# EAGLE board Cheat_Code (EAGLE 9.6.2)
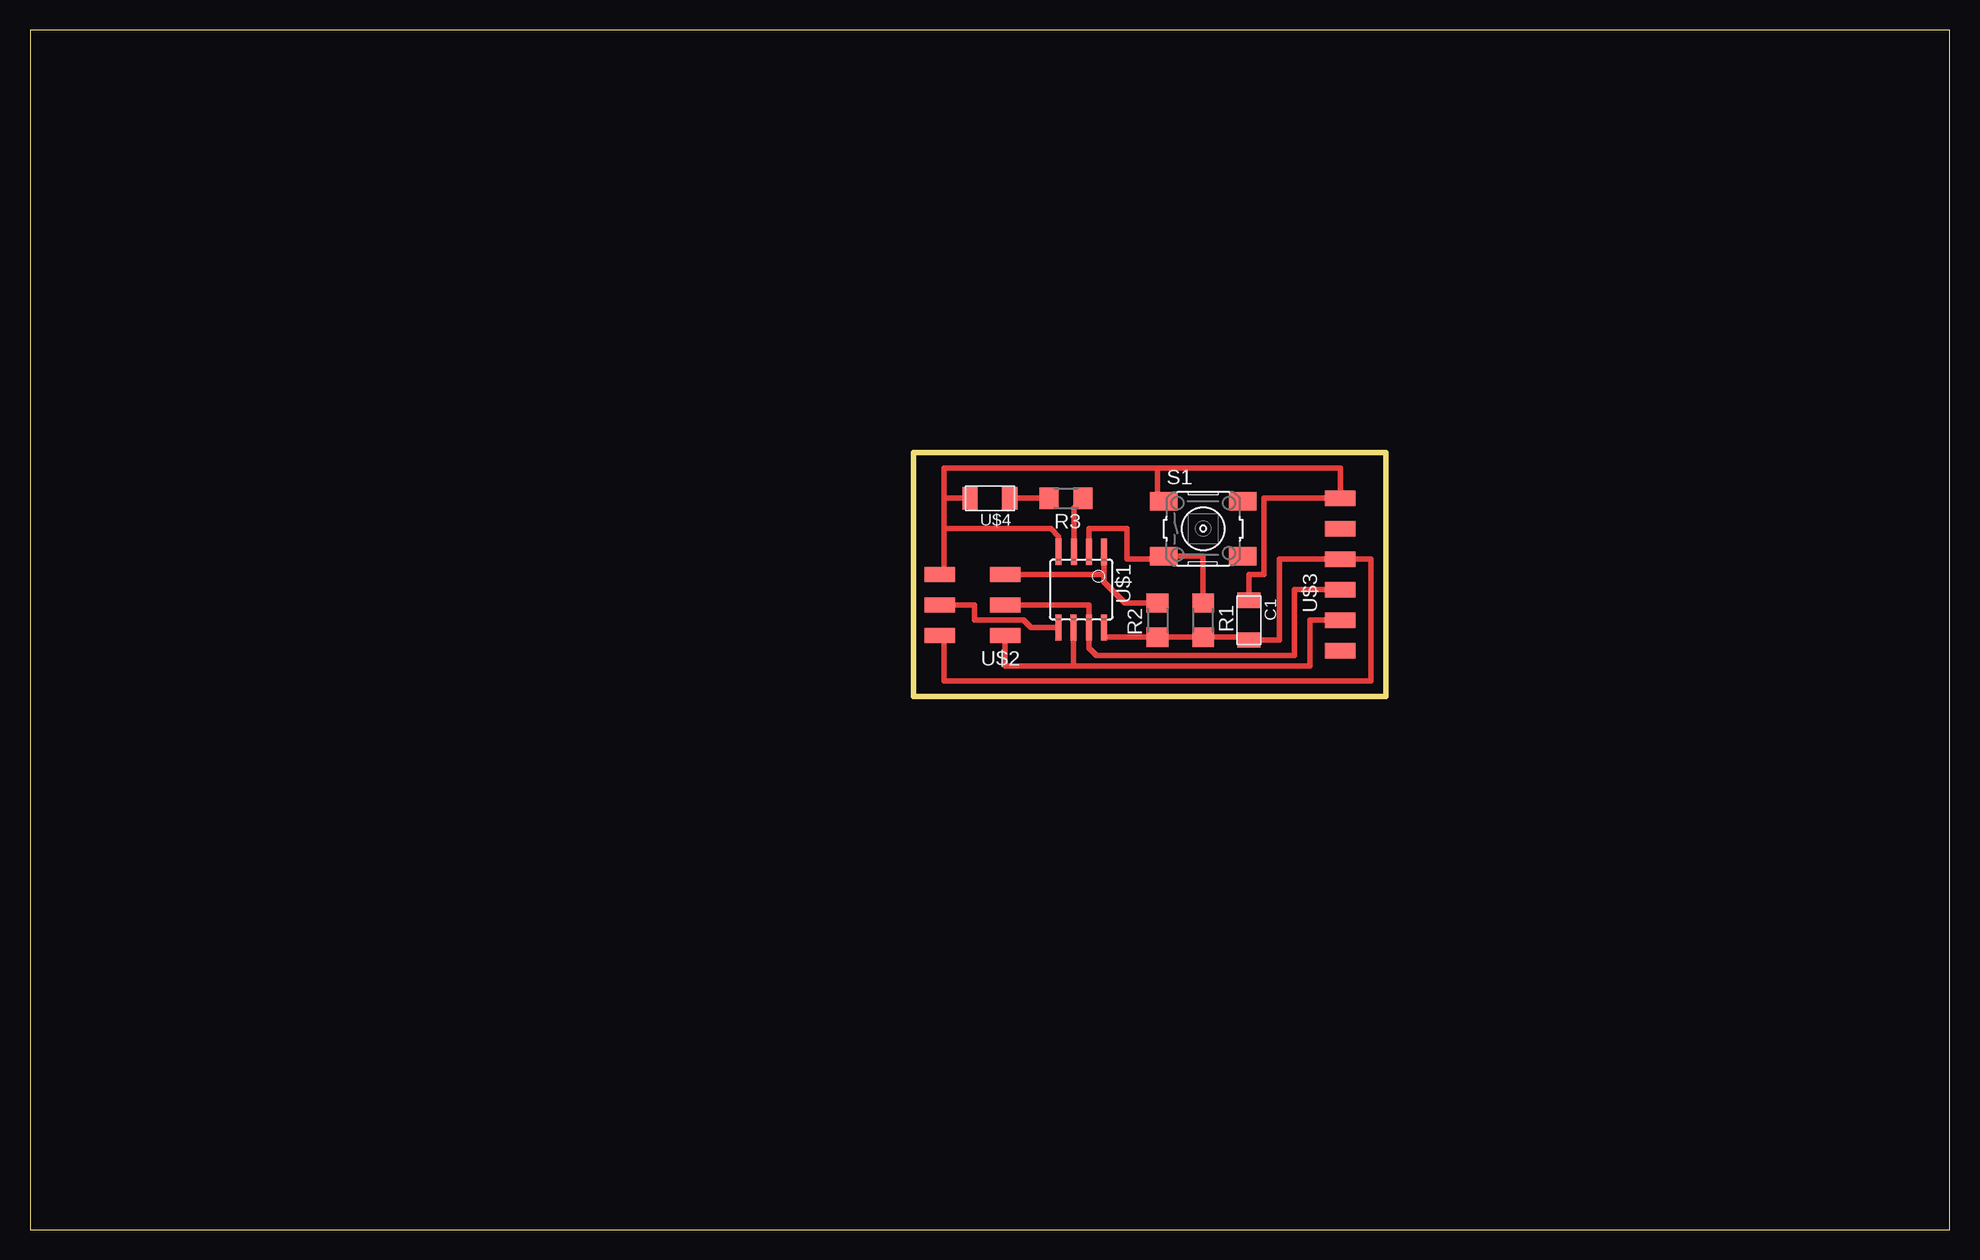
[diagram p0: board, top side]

Size 160 x 100 mm. Coordinates in mm from the lower left corner, seen from the top.
Outline: 0,0 160,0 160,100 0,100 0,0
Copper layers (1*16): Top 0.035mm / dielectric 1.5mm / Bottom 0.035mm
Design rules "default *": minimum track width 18mil, minimum drill 0.35mm, track to track 16mil, track to pad 16mil, pad to pad 16mil, via to via 12mil, smd to smd 10mil, copper to edge 40mil, drill to drill 6mil, minimum pad ring 10mil, minimum via ring 8mil, stop-mask expansion 4mil, vias tented up to drill 0mil, thermal gap 10mil
Milling: 6 lines

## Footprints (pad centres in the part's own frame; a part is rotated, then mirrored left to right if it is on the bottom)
C1206FAB = smd 1.27 x 1.905: 1 -1.651,0; 2 1.651,0
R1206 = smd 1.6 x 1.803: 1 -1.422,0; 2 1.422,0
6MM_SWITCH = smd 2.286 x 1.524: 1 -3.302,2.286; 2 3.302,2.286; 3 -3.302,-2.286; 4 3.302,-2.286
SOIC8 = smd 0.5 x 2.2: 1 -1.905,-3.154; 2 -0.645,-3.154; 3 0.625,-3.154; 4 1.895,-3.154; 5 1.905,3.154; 6 0.635,3.154; 7 -0.635,3.154; 8 -1.905,3.154
2X03SMD = smd 2.54 x 1.27: 1 -2.54,2.54; 2 2.92,2.54; 3 -2.54,0; 4 2.92,0; 5 -2.54,-2.54; 6 2.92,-2.54
1X06SMD = smd 2.54 x 1.27: 1 0,6.35; 2 0,3.81; 3 0,1.27; 4 0,-1.27; 5 0,-3.81; 6 0,-6.35
LED1206FAB = smd 1.27 x 1.905: 1 -1.651,0; 2 1.651,0

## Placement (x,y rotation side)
C1  1u  [C1206FAB]  101.6,50.8 270 top
R1  10k  [R1206]  97.79,50.8 270 top
R2  10k  [R1206]  93.98,50.8 90 top
R3  10k  [R1206]  86.36,60.96 180 top
S1  [6MM_SWITCH]  97.79,58.42 0 top
U$1  UC_ATTINY45SI  [SOIC8]  87.63,53.34 180 top
U$2  CONN_03X2_AVRISPSMD  [2X03SMD]  78.74,52.07 180 top
U$3  CONN_06_FTDI-SMD-HEADER  [1X06SMD]  109.22,54.61 0 top
U$4  LEDFAB1206  [LED1206FAB]  80.01,60.96 180 top

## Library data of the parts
C1 R1-R3 S1 U$1-U$4 = fab

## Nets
GND: C1.1 S1.1 U$1.4 U$2.6 U$3.1 U$4.2
LED: R3.1 U$1.3
N$1: U$1.6 U$2.1 U$3.5
N$2: U$1.7 U$2.3 U$3.4
N$3: R2.2 U$1.1 U$2.5
N$4: U$1.5 U$2.4
N$5: R3.2 U$4.1
PB: R1.1 S1.3 U$1.2
VCC: C1.2 R1.2 R2.1 U$1.8 U$2.2 U$3.3

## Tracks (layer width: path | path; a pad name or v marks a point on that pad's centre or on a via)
GND
  Top 0.457: 93.98,63.5 76.2,63.5 76.2,60.96 | 93.98,63.5 109.22,63.5 U$3.1 102.87,60.96 102.87,54.61 101.6,54.61 C1.1 | U$4.2 76.2,60.96 | S1.1 93.98,61.21 93.98,63.5 | U$1.4 85.73,57.77 85.09,58.42 76.2,58.42 | U$2.6 76.2,54.99 76.2,58.42 | 76.2,58.42 76.2,60.96
LED
  Top 0.457: R3.1 87,60.18 U$1.3
N$1
  Top 0.457: U$3.5 106.68,50.8 106.68,46.99 87,46.99 | 87,46.99 81.28,46.99 U$2.1 | U$1.6 87,46.99
N$2
  Top 0.457: U$3.4 105.41,53.34 105.41,47.85 88.9,47.85 88.27,48.49 U$1.7 88.27,52.07 U$2.3
N$3
  Top 0.457: U$1.1 89.53,54.61 | 89.53,54.61 89.53,53.98 91.29,52.22 R2.2 | U$2.5 89.53,54.61
N$4
  Top 0.457: U$2.4 78.74,52.07 78.74,50.8 82.81,50.8 83.43,50.19 U$1.5
N$5
  Top 0.457: U$4.1 R3.2
PB
  Top 0.457: U$1.2 88.28,58.42 91.44,58.42 91.44,55.88 94.23,55.88 S1.3 97.79,56.13 R1.1
VCC
  Top 0.457: U$2.2 76.2,49.15 76.2,45.72 111.76,45.72 111.76,55.88 U$3.3 104.14,55.88 104.14,49.15 C1.2 101.37,49.38 R1.2 R2.1 89.69,49.38 89.53,49.53 U$1.8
